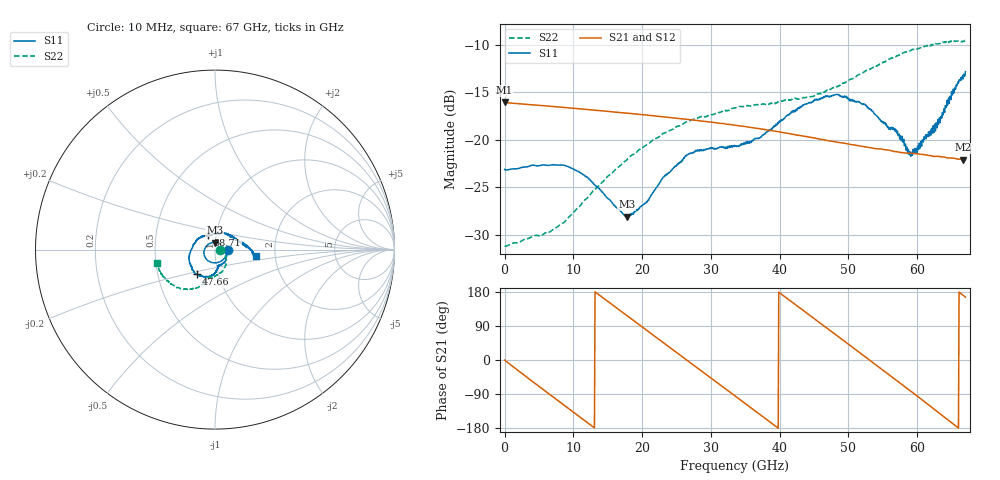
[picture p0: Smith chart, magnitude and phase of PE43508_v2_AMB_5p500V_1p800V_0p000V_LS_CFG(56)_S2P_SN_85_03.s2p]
!Keysight Technologies,N5227A,US51270237,A.10.43.00
!Date: Wednesday, August 22, 2018 17:12:26
!Correction: S11(Full 2 Port(1,3))
!S31(Full 2 Port(1,3))
!S13(Full 2 Port(1,3))
!S33(Full 2 Port(1,3))
!S2P File: Measurements: S11, S31, S13, S33:
# Hz S  dB  R 50
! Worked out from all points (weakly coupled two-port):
!   801 points, 10 MHz to 67 GHz, reference 50 ohm
!   highest |S21| = -16.05 dB at 10 MHz (marker M1); lowest = -22.1 dB at 66.67 GHz (marker M2)
!   lowest |S11| = -28.1 dB at 17.76 GHz (marker M3), VSWR 1.08, Z = 49.7 + j3.91 ohm
!   |S11| at or under -10 dB: start of sweep to end of sweep
!   |S22| runs from -31.2 to -9.5 dB; largest |S21 - S12| = 0.00071
!   S11 on the Smith chart (normalised r, x): 10 MHz: 1.15, -0.00; 47.66 GHz: 0.79, -0.22; 58.71 GHz: 0.91, +0.15; 67 GHz: 1.58, -0.12
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1e7  -23.10 -0.6  -16.05 -0.2  -16.05 -0.2  -31.17 -0.6
2.522125e9  -22.90 -40.0  -16.22 -35.5  -16.22 -35.5  -30.63 -6.1
5.787888e9  -22.66 -86.1  -16.41 -80.3  -16.41 -80.3  -29.86 -10.7
1.123082e10  -23.56 -155.9  -16.75 -154.3  -16.75 -154.2  -26.69 -18.7
1.432911e10  -25.60 160.2  -16.95 163.9  -16.95 163.9  -24.39 -26.5
1.776235e10  -28.10 92.7  -17.18 117.6  -17.18 117.6  -22.12 -38.2
2.060942e10  -26.54 32.5  -17.39 79.2  -17.39 79.2  -20.56 -48.0
2.236791e10  -24.72 1.8  -17.52 55.5  -17.52 55.5  -19.70 -54.8
2.739216e10  -21.34 -50.1  -17.90 -12.2  -17.91 -12.2  -17.84 -71.4
3.057419e10  -20.94 -69.5  -18.19 -55.2  -18.19 -55.2  -17.28 -81.5
3.3505e10  -20.64 -78.7  -18.46 -94.9  -18.46 -94.8  -16.64 -89.2
3.911541e10  -18.72 -85.7  -19.05 -170.8  -19.06 -170.6  -16.18 -99.3
4.472582e10  -16.00 -108.8  -19.75 113.1  -19.74 113.2  -15.44 -105.8
4.765664e10  -15.33 -126.7  -20.15 73.5  -20.14 73.4  -14.56 -108.1
5.234594e10  -16.25 -161.5  -20.73 9.7  -20.71 9.6  -12.81 -113.8
5.586291e10  -18.87 158.2  -21.07 -38.4  -21.07 -38.8  -11.51 -123.7
5.703524e10  -19.29 146.2  -21.25 -54.5  -21.25 -54.6  -11.13 -127.6
5.870999e10  -21.00 116.4  -21.39 -77.1  -21.40 -77.3  -10.71 -133.0
6.004979e10  -20.65 83.5  -21.46 -95.9  -21.48 -96.1  -10.44 -138.0
6.256191e10  -18.33 37.8  -21.73 -130.9  -21.75 -131.1  -9.93 -147.9
6.666505e10  -13.58 -6.3  -22.10 170.8  -22.16 170.9  -9.59 -164.6
6.7e10  -12.82 -9.3  -22.08 166.0  -22.16 166.0  -9.56 -166.5
